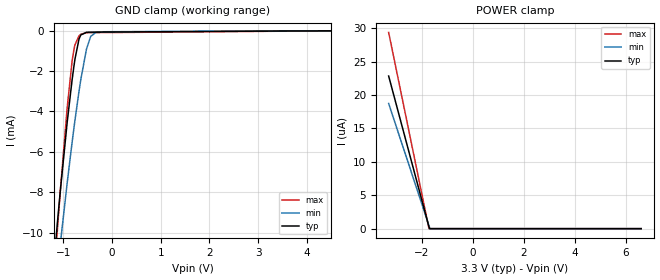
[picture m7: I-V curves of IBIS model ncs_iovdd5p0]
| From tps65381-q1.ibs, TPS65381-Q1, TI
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|   ncs_iovdd5p0 Model
[Model]   ncs_iovdd5p0
Model_type   Input
Vinl = 0.99
Vinh = 2.31
|   typ   min   max
|   (nom PVT)   (fast PVT)   (slow PVT)
C_comp   8.028e-13   7.804e-13   8.085e-13
[Model spec]
|subparameter
Vinl   0.99   0.951   1.029
Vinh   2.31   2.219   2.401
| Where nom  PVT is Nominal Process, 3.3V, 27C
|   Fast PVT is Strong Process,  3.43V, -40C
|   Slow PVT is Weak Process,   3.17V, 150C
[Voltage Range]   3.3   3.17   3.43
|Junction Temperature
[Temperature Range]   27   150   -40
[Power Clamp Reference]   3.3   3.17   3.43
[GND Clamp Reference]   0   0   0
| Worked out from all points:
|   GND clamp passes 1 mA (typ) near -0.73 V on its own axis
[GND Clamp]
|   Voltage   I(typ)   I(min)   I(max)
-3.3V     -92.26mA   -77.05mA   -111.9mA
-1.228V   -12.46mA   -14.38mA   -13.46mA
-1.119V   -9.464mA   -11.86mA   -9.8mA
-1.059V   -7.901mA   -10.52mA   -7.892mA
-923mV    -4.613mA   -7.606mA   -3.917mA
-820.1mV  -2.465mA   -5.555mA   -1.537mA
-758.4mV  -1.387mA   -4.404mA   -693.6uA
-640.2mV  -217.8uA   -2.427mA   -179.2uA
-523.1mV  -83.42uA   -906.4uA   -108.3uA
-437.5mV  -77.95uA   -290.6uA   -104uA
-301.2mV  -75.68uA   -72.45uA   -101.3uA
6.6V      0A         0A         0A
[POWER Clamp]
|   Voltage   I(typ)   I(min)   I(max)
-3.3V     22.84uA    18.73uA    29.37uA
-1.715V   219.1nA    413.2nA    0A
-1.703V   40.08nA    268.2nA    0A
-1.68V    0A         0A         0A
6.6V      0A         0A         0A
